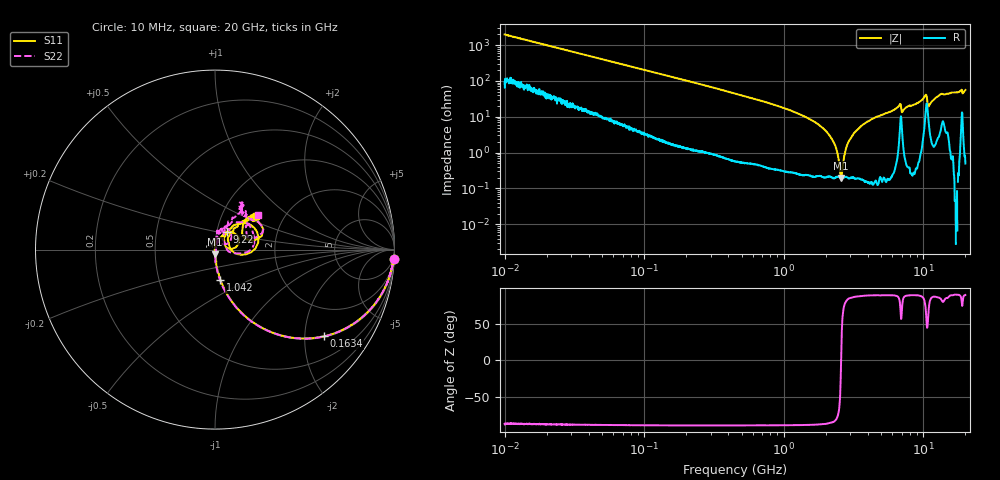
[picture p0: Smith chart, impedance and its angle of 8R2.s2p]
!Keysight Technologies,P5008B,MY61100088,A.16.20.02
!Date: Friday, August 30, 2024 13:20:26
!Correction: S11(C  2-Port  )
!S21(C  2-Port  )
!S12(C  2-Port  )
!S22(C  2-Port  )
!S2P File: Measurements: S11, S21, S12, S22:Log Frequency Sweep
# Hz S  dB  R 50
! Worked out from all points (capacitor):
!   1601 points, 10 MHz to 20 GHz, reference 50 ohm
!   read as one part in series: C = 8.08 pF near 10.39 MHz
!   lowest |Z| = 195 mohm at 2.569 GHz (marker M1)
!   series resonance near 2.574 GHz, so ESL is about 470 pH
!   S11 on the Smith chart (normalised r, x): 10 MHz: 2, -39; 163.4 MHz: 1.03, -2.49; 1.042 GHz: 1.00, -0.35; 9.22 GHz: 1.12, +0.23; 20 GHz: 1.45, +0.60
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1e7  -0.03 -2.9  -25.93 84.4  -25.93 84.4  -0.03 -2.9
3.555162e7  -0.18 -10.0  -15.19 78.3  -15.20 78.3  -0.18 -10.1
1.263918e8  -1.47 -31.7  -5.62 57.5  -5.62 57.5  -1.47 -31.8
1.633535e8  -2.21 -38.6  -4.14 50.7  -4.15 50.7  -2.21 -38.6
4.472136e8  -7.76 -65.5  -0.85 23.7  -0.85 23.7  -7.76 -65.8
1.041729e9  -15.27 -79.8  -0.16 8.9  -0.16 8.8  -15.28 -80.7
1.589917e9  -20.58 -84.2  -0.06 3.7  -0.06 3.7  -20.56 -85.8
2.568928e9  -31.60 -86.6  -0.02 -1.5  -0.02 -1.5  -31.32 -87.7
2.838428e9  -37.88 -92.5  -0.01 -2.6  -0.02 -2.6  -36.72 -74.1
3.166141e9  -54.69 141.3  -0.01 -3.8  -0.02 -3.9  -44.21 -3.9
3.304445e9  -45.05 81.9  -0.01 -4.3  -0.02 -4.4  -44.99 42.7
3.548507e9  -35.89 86.3  -0.01 -5.2  -0.01 -5.2  -36.14 66.7
3.774562e9  -32.33 97.6  -0.01 -6.0  -0.01 -6.0  -32.56 60.9
4.436224e9  -27.49 85.4  -0.02 -8.1  -0.02 -8.1  -27.64 74.0
5.652411e9  -24.12 74.7  -0.02 -11.8  -0.02 -11.9  -23.70 76.3
6.674885e9  -18.74 53.1  -0.18 -16.3  -0.18 -16.4  -18.80 75.0
7.236311e9  -22.64 46.0  -0.09 -14.3  -0.09 -14.4  -23.39 85.1
9.220141e9  -18.49 56.9  -0.07 -22.2  -0.08 -22.4  -18.53 70.7
1.028466e10  -12.66 38.1  -0.87 -29.1  -0.88 -29.3  -12.95 42.6
1.12028e10  -21.11 34.9  -0.24 -22.3  -0.24 -22.4  -22.64 54.0
1.329228e10  -11.38 41.9  -0.60 -32.0  -0.60 -32.1  -11.69 55.5
2e10  -10.57 39.6  -0.42 -49.6  -0.42 -49.8  -10.30 38.8
